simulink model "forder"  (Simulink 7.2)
settings: Solver=ode45  StartTime=0.0  StopTime=10.0  RelTol=1e-3
libraries: simulink x1

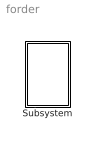
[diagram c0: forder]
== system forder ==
  Subsystem : Subsystem

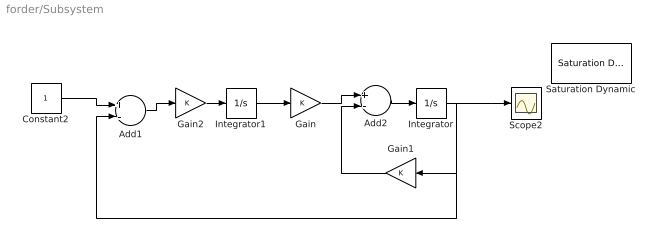
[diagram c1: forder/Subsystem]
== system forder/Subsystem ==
  Add1 : Sum  Inputs=+-  OutDataType=sfix(16)  OutScaling=2^-10
  Add2 : Sum  Inputs=+-  OutDataType=sfix(16)  OutScaling=2^-10
  Constant2 : Constant  OutDataType=sfix(16)  OutScaling=2^0
  Gain : Gain  ParameterDataType=sfix(16)  ParameterScaling=2^0  OutDataType=sfix(16)  OutScaling=2^0
  Gain1 : Gain  Orientation=left  ParameterDataType=sfix(16)  ParameterScaling=2^0  OutDataType=sfix(16)  OutScaling=2^0
  Gain2 : Gain  ParameterDataType=sfix(16)  ParameterScaling=2^0  OutDataType=sfix(16)  OutScaling=2^0
  Integrator : Integrator
  Integrator1 : Integrator
  Saturation Dynamic : simulink/Discontinuities/Saturation Dynamic  SystemSampleTime=-1  OutMin=[]  OutMax=[]  OutDataTypeStr=Inherit: Same as second input  OutDataType=sfix(16)  OutScaling=2^-10  DoSatur=off
  Scope2 : Scope
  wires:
  Constant2/1 -> Add1/1
  Integrator/1 -> Scope2/1, Gain1/1, Add1/2
  Gain1/1 -> Add2/2
  Gain/1 -> Add2/1
  Add2/1 -> Integrator/1
  Integrator1/1 -> Gain/1
  Gain2/1 -> Integrator1/1
  Add1/1 -> Gain2/1
